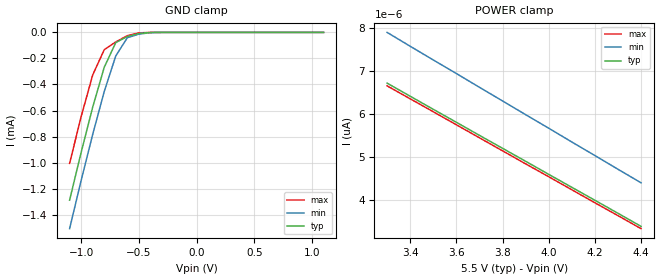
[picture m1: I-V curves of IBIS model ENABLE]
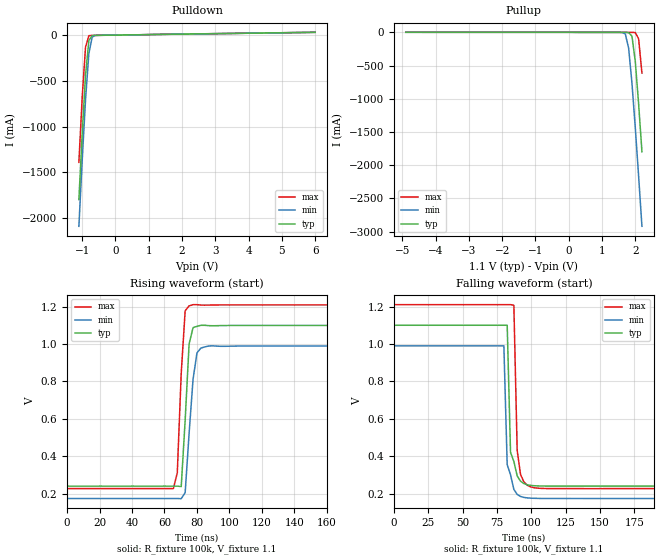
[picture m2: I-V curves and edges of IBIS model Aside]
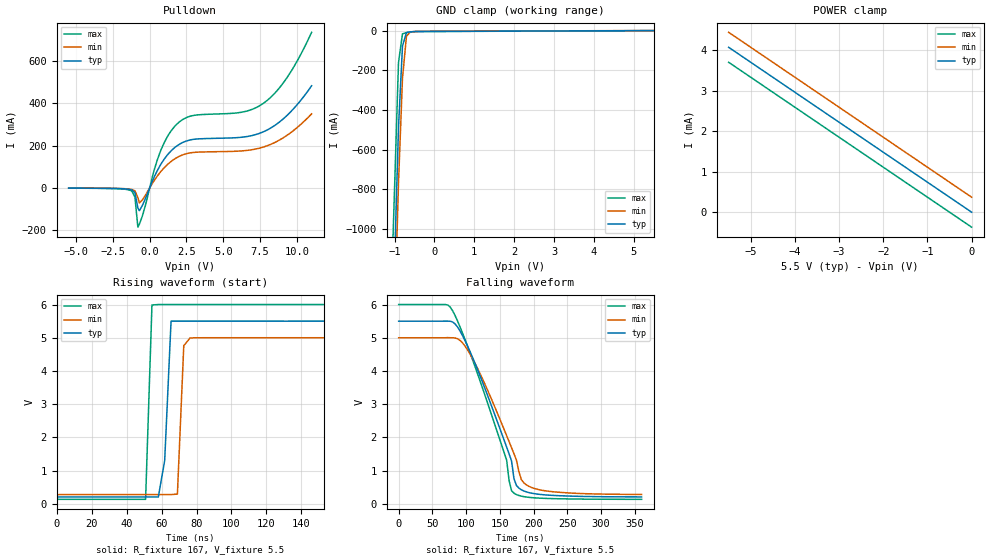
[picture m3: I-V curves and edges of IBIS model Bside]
| PCA9519 - IBIS model
| Note on Port A behavior:
| Since port A (low voltage side) has an internal pull up current source and a
| 200 ohm pull down driver as documented in the datasheet, the pull down curve
| will have a nearly linear behavior since the pull down is dominated by the
| 200ohm resistive path.
[IBIS Ver]   4.0
[Comment Char]   |_char
| Aside = 1.1V Bside = 5.5V
[File name]   pca9519_a1_1b_5_5.ibs
[File Rev]   1
[Date]   Sept 23, 2009 3:54:05 PM
[Source]
[Notes]
|The package model information is simulated at 400 kHz,
|which is the maximum system operating frequency.
[Disclaimer]
(C) Copyright 2007 NXP Semiconductors
All rights reserved
NXP Semiconductors (NXP) does not warrant that this model and any other
accompanying information (Model) accurately or fully represents the
operating characteristics and specifications of the semiconductor
products to which the Model relates.  Moreover, the Model is furnished
on an "as is" and with "all faults" basis, and without support or
warranty of any kind.  NXP disclaims all warranties, whether expressed
or implied or statutory, including without limitation all implied
warranties of non-infringement, merchantability and fitness for any
purpose, and those arising from a course of dealing or usage of trade.
NXP does not convey any license under its or any third party's patents,
copyrights or other intellectual property or proprietary rights.
You and your company assume any and all risks and liability arising out
of the application or use of the Model.
In no event shall NXP be liable for any direct, indirect, special,
consequential or incidental damages, however caused, whether in
warranty, contract or tort (including negligence), strict liability or
other legal theory, including, without limitation, for lost profits,
business interruption, or corruption or loss of data or information,
arising out of or in connection with the use of or the inability to use
the Model, even if NXP has been advised of the possibility of such
damages.
NXP provides the Model as a courtesy to our customers. You and your
company shall not distribute, convey, sell, or give the Model to anyone
else without receiving prior written permission from NXP.
NXP reserves the right to make changes without notice to the Model to
improve reliability, function, or design.
Please be aware that your receipt and subsequent use of the Model shall
serve as acceptance of these terms and conditions.  If you do not
accept these terms, return or destroy the Model immediately.
[Copyright]
(C) Copyright 2009 NXP Semiconductors  All rights reserved
| HVQFN24 - package
[Component]   PCA9519BS
Si_location Die
Timing_location Pin
[Manufacturer]   NXP Semiconductors
[Package]
|variable   typ   min   max
R_pkg   3.74E-03   3.16E-03   4.32E-03
L_pkg   1.22E-09   0.99E-09   1.45E-09
C_pkg   0.20E-12   0.18E-12   0.22E-12
[Pin] signal_name   model_name   R_pin   L_pin   C_pin
1   A2   Aside   4.32E-03  1.45E-09  0.22E-12
2   A3   Aside   3.88E-03  1.27E-09  0.21E-12
3   A4   Aside   3.68E-03  1.18E-09  0.20E-12
4   A5   Aside   3.68E-03  1.18E-09  0.20E-12
5   A6   Aside   3.88E-03  1.26E-09  0.21E-12
6   A7   Aside   4.30E-03  1.44E-09  0.22E-12
7   A8   Aside   4.15E-03  1.40E-09  0.21E-12
8   NC   NC   NA   NA   NA
9   NC   NC   NA   NA   NA
10   VCCB   POWER   3.16E-03  0.99E-09  0.18E-12
11   EN   ENABLE   3.31E-03  1.06E-09  0.19E-12
12   B8   Bside   4.15E-03  1.39E-09  0.22E-12
13   B7   Bside   4.33E-03  1.45E-09  0.22E-12
14   B6   Bside   3.90E-03  1.27E-09  0.21E-12
15   B5   Bside   3.69E-03  1.18E-09  0.20E-12
16   B4   Bside   3.68E-03  1.18E-09  0.20E-12
17   B3   Bside   3.88E-03  1.26E-09  0.21E-12
18   B2   Bside   4.29E-03  1.44E-09  0.22E-12
19   B1   Bside   4.12E-03  1.39E-09  0.21E-12
20   NC   NC   NA   NA   NA
21   NC   NC   NA   NA   NA
22   GND   GND   3.20E-03  1.01E-09  0.18E-12
23   VCCA   POWER   3.37E-03  1.08E-09  0.19E-12
24   A1   Aside   4.12E-03  1.38E-09  0.21E-12
[Package Model]   hvqfn24_sot616ac2
|The package model information is simulated at 400 kHz,
|which is the maximum system operating frequency.
| TSSOP8 - package
[Component]   PCA9519PW
Si_location Die
Timing_location Pin
[Manufacturer]   NXP Semiconductors
[Package]
|variable   typ   min   max
R_pkg   4.66E-03   4.03E-03   5.28E-03
L_pkg   2.39E-09   1.87E-09   2.90E-09
C_pkg   0.36E-12   0.30E-12   0.42E-12
[Pin] signal_name   model_name   R_pin   L_pin   C_pin
1   EN   ENABLE   4.30E-03  2.79E-09  0.42E-12
2   B1   Bside   4.95E-03  2.58E-09  0.41E-12
3   B2   Bside   5.28E-03  2.39E-09  0.35E-12
4   B3   Bside   4.59E-03  2.08E-09  0.32E-12
5   B4   Bside   4.04E-03  1.87E-09  0.30E-12
6   B5   Bside   4.03E-03  1.87E-09  0.30E-12
7   B6   Bside   4.57E-03  2.07E-09  0.32E-12
8   B7   Bside   5.26E-03  2.38E-09  0.35E-12
9   B8   Bside   4.87E-03  2.56E-09  0.41E-12
10   GND   GND   4.39E-03  2.85E-09  0.42E-12
11   VCCA   POWER   4.33E-03  2.81E-09  0.42E-12
12   A8   Aside   4.88E-03  2.56E-09  0.41E-12
13   A7   Aside   5.28E-03  2.38E-09  0.35E-12
14   A6   Aside   4.56E-03  2.07E-09  0.32E-12
15   A5   Aside   4.03E-03  1.87E-09  0.30E-12
16   A4   Aside   4.04E-03  1.88E-09  0.30E-12
17   A3   Aside   4.58E-03  2.09E-09  0.32E-12
18   A2   Aside   5.28E-03  2.39E-09  0.35E-12
19   A1   Aside   4.91E-03  2.57E-09  0.41E-12
20   VCCB   POWER   4.46E-03  2.90E-09  0.42E-12
[Package Model]   tssop20_sot360db7
|   PACKAGE MODEL HVQFN24
[Define Package Model]   hvqfn24_sot616ac2
[Manufacturer]  NXP
[OEM]  NXP
[Description]   Full package IBIS model.Simulated @ 400kHz
[Number Of Pins]  20
[Pin Numbers]
|Pin Num   Terminal Name
1   | Lead1:pin1
2   | Lead2:pin2
3   | Lead3:pin3
4   | Lead4:pin4
5   | Lead5:pin5
6   | Lead6:pin6
7   | Lead7:pin7
8   | Lead10:pin8
9   | Lead11:pin9
10   | Lead12:pin10
11   | Lead13:pin11
12   | Lead14:pin12
13   | Lead15:pin13
14   | Lead16:pin14
15   | Lead17:pin15
16   | Lead18:pin16
17   | Lead19:pin17
18   | Lead22:pin18
19   | Lead23:pin19
20   | Lead24:pin20
[Model Data]
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[End Model Data]
[End Package Model]
|   PACKAGE MODEL TSSOP20
[Define Package Model]  tssop20_sot360db7
[Manufacturer]  NXP
[OEM] NXP
[Description]   Full package IBIS model.Simulated @ 400kHz
[Number Of Pins]  20
[Pin Numbers]
|Pin Num   Terminal Name
1   | Lead1:pin1
2   | Lead2:pin2
3   | Lead3:pin3
4   | Lead4:pin4
5   | Lead5:pin5
6   | Lead6:pin6
7   | Lead7:pin7
8   | Lead8:pin8
9   | Lead9:pin9
10   | Lead10:pin10
11   | Lead11:pin11
12   | Lead12:pin12
13   | Lead13:pin13
14   | Lead14:pin14
15   | Lead15:pin15
16   | Lead16:pin16
17   | Lead17:pin17
18   | Lead18:pin18
19   | Lead19:pin19
20   | Lead20:pin20
[Model Data]
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[End Model Data]
[End Package Model]
| Models and submodels in the file (3): ENABLE (Input), Aside (I/O), Bside (I/O_open_drain)
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|The package model information is simulated at 400 kHz,
|which is the maximum system operating frequency.
[Model]   ENABLE
Model_type Input
Vinh=5
Vinl=1
|variable   typ   min   max
C_comp   1.84p   1.81p   1.86p
[Temperature Range] 27   85   -40
[Voltage Range]   5.5   5   6
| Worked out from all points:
|   GND clamp passes 1 mA (typ) near -1.02 V on its own axis
[GND Clamp]
-1.1V     -1.288mA   -1.507mA   -1.005mA
-1V       -921.3uA   -1.137mA   -647uA
-900mV    -574.4uA   -783.6uA   -327uA
-800mV    -268uA     -454.2uA   -133.1uA
-700mV    -78.19uA   -180.8uA   -72.93uA
-600mV    -31.83uA   -40.83uA   -25.26uA
-500mV    -8.452uA   -13.3uA    -3.68uA
-400mV    -758.4nA   -2.213uA   -96.83nA
1.1V      3.384pA    4.4pA      3.331pA
[POWER Clamp]
3.3V      6.725pA    7.908pA    6.661pA
3.4V      6.42pA     7.585pA    6.359pA
3.5V      6.114pA    7.265pA    6.057pA
3.6V      5.812pA    6.949pA    5.754pA
3.7V      5.507pA    6.628pA    5.45pA
3.8V      5.205pA    6.31pA     5.146pA
3.9V      4.903pA    5.99pA     4.842pA
4V        4.597pA    5.674pA    4.542pA
4.1V      4.295pA    5.352pA    4.238pA
4.2V      3.993pA    5.036pA    3.935pA
4.3V      3.689pA    4.716pA    3.634pA
4.4V      3.384pA    4.4pA      3.331pA
[Model]   Aside
Model_type I/O
Enable Active-High
Vinh=0.7
Vinl=0.2
Vref=1.1
Vmeas=0.55
Rref=100k
Cref=20p
|variable   typ   min   max
C_comp   8.4p   8.2p   8.6p
[Model Spec]
Vinh   0.77   0.7   1.21
Vinl   0.15   0.15   0.3
[Temperature Range] 27   85   -40
[Voltage Range]   1.1   0.99   1.21
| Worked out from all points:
|   slope of the pulldown table from 0 to 0.165 V, typ, clamps not added: 202 ohm
|   slope of the pullup table from 0 to 0.165 V, typ, clamps not added: 283 ohm
|   falling waveform, R_fixture 100k, V_fixture 1.1: 20-80 % time 2.26ns typ, 2.63ns min, 1.97ns max; typ from 1.1 V to 0.24 V
|   rising waveform, R_fixture 100k, V_fixture 1.1: 20-80 % time 3.23ns typ, 4.11ns min, 3.14ns max; typ from 0.24 V to 1.1 V
[Pullup]
-4.9V     64.41uA    62.23uA    71.57uA
1.5V      -1.236mA   -1.234mA   -1.146mA
1.6V      -1.417mA   -2.775mA   -1.157mA
1.7V      -1.759mA   -25.04mA   -1.249mA
1.8V      -4.058mA   -238.2mA   -1.518mA
1.9V      -58.77mA   -766.2mA   -1.883mA
2V        -438.6mA   -1.437A    -3.917mA
2.1V      -1.076A    -2.164A    -98.36mA
2.2V      -1.798A    -2.92A     -613.2mA
[Pulldown]
-1.1V     -1.798A    -2.09A     -1.391A
-1V       -1.076A    -1.367A    -679.7mA
-900mV    -439.5mA   -705.3mA   -132.5mA
-800mV    -60.9mA    -201.9mA   -7.696mA
-700mV    -6.598mA   -21.62mA   -4.639mA
-600mV    -4.181mA   -4.679mA   -4.12mA
-500mV    -3.643mA   -3.295mA   -3.621mA
6V        29.24mA    28.83mA    29.58mA
[Falling Waveform]
R_fixture=100k
V_fixture=1.1
V_fixture_min=0.99
V_fixture_max=1.21
0s        1.1V       990mV      1.21V
80ns      1.1V       989.9mV    1.21V
82.42ns   1.1V       355.2mV    1.21V
84.85ns   421.1mV    301.2mV    1.21V
87.27ns   372.6mV    223mV      1.206V
89.7ns    294.9mV    196.2mV    431.9mV
92.12ns   267.1mV    185.5mV    302.7mV
96.97ns   247.9mV    177.6mV    245.9mV
111.5ns   240.8mV    174.5mV    227.6mV
240ns     240.1mV    173.4mV    227.2mV
[Rising Waveform]
R_fixture=100k
V_fixture=1.1
V_fixture_min=0.99
V_fixture_max=1.21
0s        239.8mV    173.4mV    226.6mV
65.45ns   239.8mV    173.4mV    226.6mV
67.88ns   239.8mV    173.4mV    311mV
70.3ns    237.4mV    172.6mV    844.6mV
72.73ns   593mV      205.1mV    1.178V
75.15ns   1.001V     521.9mV    1.205V
77.58ns   1.088V     811.1mV    1.211V
80ns      1.095V     953.5mV    1.211V
82.42ns   1.101V     978.7mV    1.209V
240ns     1.1V       990mV      1.21V
[Ramp]
R_load=100k
dV/dt_r   5.112E-1/2.618E-9   4.849E-1/3.941E-9   5.855E-1/2.900E-9
dV/dt_f   5.160E-1/2.423E-9   4.900E-1/2.388E-9   5.897E-1/2.355E-9
|[End   Aside
[Model]   Bside
Model_type I/O_open_drain
Enable Active-High
Vinh=5
Vinl=1
Vref=5.5
Vmeas=2.75
Rref=167
Cref=57p
|variable   typ   min   max
C_comp   7.72p   7.7p   7.74p
[Model Spec]
Vinh   3.85   3.5   5.5
Vinl   1.65   1.5   1.8
[Temperature Range] 27   85   -40
[Voltage Range]   5.5   5   6
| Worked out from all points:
|   slope of the pulldown table from 0 to 0.825 V, typ, clamps not added: 6.92 ohm
|   POWER clamp passes 1 mA (typ) near -1.35 V on its own axis
|   falling waveform, R_fixture 167, V_fixture 5.5: 20-80 % time 58.7ns typ, 58.1ns min, 59.5ns max; typ from 5.5 V to 0.209 V
|   rising waveform, R_fixture 167, V_fixture 5.5: 20-80 % time 2.84ns typ, 2.31ns min, 2.19ns max; typ from 0.206 V to 5.5 V
[Pulldown]
-5.5V     -773uA     -642uA     -963uA
-1.3V     -7.933mA   -5.931mA   -11.58mA
-1V       -21.34mA   -13.65mA   -43.56mA
-800mV    -94.72mA   -45.19mA   -185.1mA
-500mV    -83.34mA   -57.29mA   -133.6mA
700mV     105mA      72.72mA    167.6mA
1.7V      190.8mA    137.4mA    291.1mA
2.8V      227.8mA    166.5mA    340.1mA
6.2V      239.5mA    174.9mA    357.5mA
7.7V      264.8mA    193mA      399mA
9.3V      340.8mA    247.5mA    518.5mA
11V       482.9mA    350.2mA    735.6mA
[GND Clamp]
-5.5V     -37.88A    -38.1A     -37.57A
-1.1V     -1.864A    -2.167A    -1.444A
-900mV    -489.2mA   -768.6mA   -161.3mA
-800mV    -77.8mA    -240.2mA   -16.34mA
-700mV    -10.16mA   -27.68mA   -10.28mA
-600mV    -6.581mA   -6.541mA   -6.603mA
5.5V      267.1pA    370.4uA    -370.4uA
[POWER Clamp]
-5.5V     4.074mA    4.444mA    3.704mA
-5.2V     3.852mA    4.222mA    3.481mA
-4.1V     3.037mA    3.407mA    2.667mA
0V        267.1pA    370.4uA    -370.4uA
[Falling Waveform]
R_fixture=167
V_fixture=5.5
V_fixture_min=5
V_fixture_max=6
0s        5.5V       5V         6V
69.09ns   5.501V     5V         6.001V
80ns      5.474V     5V         5.811V
109.1ns   4.426V     4.387V     4.36V
160ns     1.708V     2.054V     1.314V
167.3ns   1.289V     1.69V      394.8mV
170.9ns   753.4mV    1.507V     321.1mV
181.8ns   422.9mV    728mV      231.6mV
200ns     309.7mV    469.2mV    183mV
360ns     208.6mV    282.3mV    135.7mV
[Rising Waveform]
R_fixture=167
V_fixture=5.5
V_fixture_min=5
V_fixture_max=6
0s        206mV      277.1mV    134.6mV
50.91ns   206mV      277.1mV    134.6mV
54.55ns   206mV      277.1mV    5.987V
58.18ns   206mV      277.1mV    5.999V
61.82ns   1.302V     277.1mV    6V
65.45ns   5.5V       277.1mV    6.001V
69.09ns   5.5V       292.9mV    6V
72.73ns   5.5V       4.762V     6V
76.36ns   5.5V       4.995V     5.999V
240ns     5.5V       5V         6V
[Ramp]
R_load=1350
dV/dt_r   1.959E+0/1.367E-9   1.770E+0/1.646E-9   2.147E+0/1.168E-9
dV/dt_f   1.956E+0/2.998E-8   1.763E+0/2.973E-8   2.146E+0/3.149E-8
|[End   Bside
